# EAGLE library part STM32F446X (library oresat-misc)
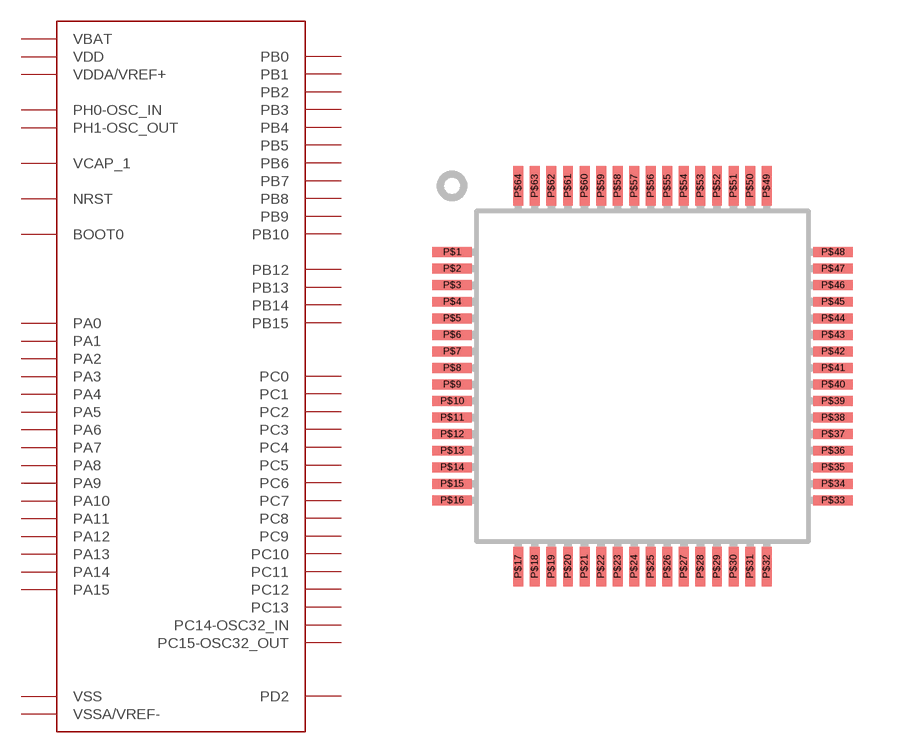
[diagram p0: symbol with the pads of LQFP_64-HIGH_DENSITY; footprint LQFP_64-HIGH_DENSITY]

Designator prefix -

## STM32F446X  [LQFP_64-HIGH_DENSITY]
P$1  VBAT  pwr
P$2  PC13
P$3  PC14-OSC32_IN
P$4  PC15-OSC32_OUT
P$5  PH0-OSC_IN
P$6  PH1-OSC_OUT
P$7  NRST
P$8  PC0
P$9  PC1
P$10  PC2
P$11  PC3
P$12  VSSA/VREF-  pwr
P$13  VDDA/VREF+  pwr
P$14  PA0
P$15  PA1
P$16  PA2
P$17  PA3
P$18  VSS  pwr
P$19  VDD  pwr
P$20  PA4
P$21  PA5
P$22  PA6
P$23  PA7
P$24  PC4
P$25  PC5
P$26  PB0
P$27  PB1
P$28  PB2
P$29  PB10
P$30  VCAP_1
P$31  VSS  pwr
P$32  VDD  pwr
P$33  PB12
P$34  PB13
P$35  PB14
P$36  PB15
P$37  PC6
P$38  PC7
P$39  PC8
P$40  PC9
P$41  PA8
P$42  PA9
P$43  PA10
P$44  PA11
P$45  PA12
P$46  PA13
P$47  VSS  pwr
P$48  VDD  pwr
P$49  PA14
P$50  PA15
P$51  PC10
P$52  PC11
P$53  PC12
P$54  PD2
P$55  PB3
P$56  PB4
P$57  PB5
P$58  PB6
P$59  PB7
P$60  BOOT0
P$61  PB8
P$62  PB9
P$63  VSS  pwr
P$64  VDD  pwr

## Footprint LQFP_64-HIGH_DENSITY (pad centres in mm)
smd 1.2 x 0.3: P$1 -5.75,3.75; P$2 -5.75,3.25; P$3 -5.75,2.75; P$4 -5.75,2.25; P$5 -5.75,1.75; P$6 -5.75,1.25; P$7 -5.75,0.75; P$8 -5.75,0.25; P$9 -5.75,-0.25; P$10 -5.75,-0.75; P$11 -5.75,-1.25; P$12 -5.75,-1.75; P$13 -5.75,-2.25; P$14 -5.75,-2.75; P$15 -5.75,-3.25; P$16 -5.75,-3.75; P$33 5.75,-3.75; P$34 5.75,-3.25; P$35 5.75,-2.75; P$36 5.75,-2.25; P$37 5.75,-1.75; P$38 5.75,-1.25; P$39 5.75,-0.75; P$40 5.75,-0.25; P$41 5.75,0.25; P$42 5.75,0.75; P$43 5.75,1.25; P$44 5.75,1.75; P$45 5.75,2.25; P$46 5.75,2.75; P$47 5.75,3.25; P$48 5.75,3.75
smd 0.3 x 1.2: P$17 -3.75,-5.75; P$18 -3.25,-5.75; P$19 -2.75,-5.75; P$20 -2.25,-5.75; P$21 -1.75,-5.75; P$22 -1.25,-5.75; P$23 -0.75,-5.75; P$24 -0.25,-5.75; P$25 0.25,-5.75; P$26 0.75,-5.75; P$27 1.25,-5.75; P$28 1.75,-5.75; P$29 2.25,-5.75; P$30 2.75,-5.75; P$31 3.25,-5.75; P$32 3.75,-5.75; P$49 3.75,5.75; P$50 3.25,5.75; P$51 2.75,5.75; P$52 2.25,5.75; P$53 1.75,5.75; P$54 1.25,5.75; P$55 0.75,5.75; P$56 0.25,5.75; P$57 -0.25,5.75; P$58 -0.75,5.75; P$59 -1.25,5.75; P$60 -1.75,5.75; P$61 -2.25,5.75; P$62 -2.75,5.75; P$63 -3.25,5.75; P$64 -3.75,5.75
